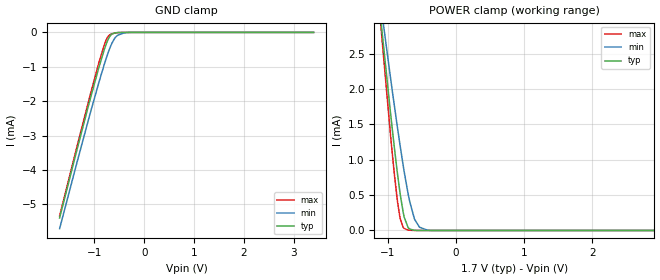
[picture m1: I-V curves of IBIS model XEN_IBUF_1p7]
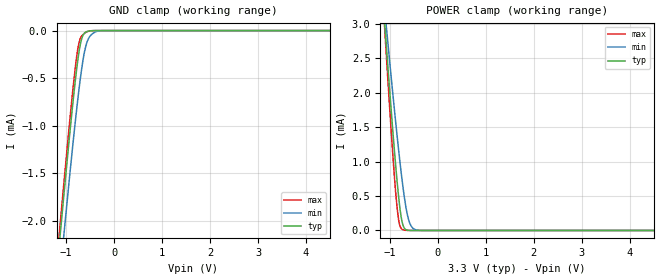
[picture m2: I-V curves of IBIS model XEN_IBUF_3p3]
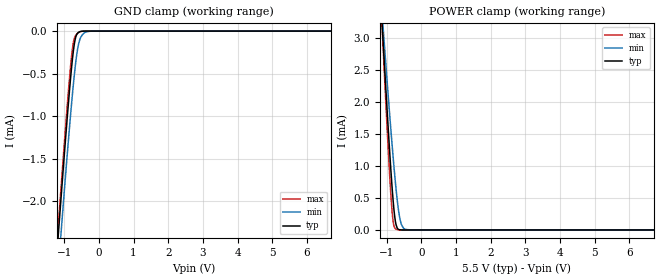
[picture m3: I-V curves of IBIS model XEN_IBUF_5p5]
|Texas Instruments Incorporated
| DAC874xH, HART & FOUNDATION Fieldbus / PROFIBUS PA Modems
| Device NAme#   Digital Voltage Range   Package-type   #pins
| DAC8740H   1.71V-5.5V   VQFN   24
| DAC8741H   1.71V-5.5V   VQFN   24
| DAC8742H   1.71V-5.5V   VQFP   32
[IBIS Ver]   4.1
[File name]   dac874xh.ibs
[Date]   02/17/2017
[File Rev]   1.0
[Source]
| Texas Instruments Incorporated.
| Analog-eLab Design Center, HPA
| 12500 TI Blvd
| Dallas, TX -75243
[Notes]   Revision History:
| Rev 1.0: 02/17/2017
| - Initial version of the model
| - Model generated from simulations in SPECTRE
| - Model matched to SPICE simulation
| - C_comp although listed in numerical order of value are
|   obtained from varying PVT conditions. For PVT conditions for
|   each specific value refer the buffer description under
|   respective [Model]. IBIS model user is responsible for using
|   appropriate C_comp to simulate for Signal Integrity.
[Disclaimer]
| This model is designed as an aid for customers of Texas Instruments.
| TI and its licensors and suppliers make no warranties, either expressed
| or implied, with respect to this  model, including the warranties of
| merchantability or fitness for a particular purpose. The model is
| provided solely on an "as is" basis. The entire risk as to its quality
| and performance is with the customer.
[Copyright]
(C) Copyright 2017 Texas Instruments Incorporated.All rights reserved.
|   DAC8740H
[Component]   DAC8740H
[Manufacturer]  TI
[Package]   |24 VQFN
|   typ   min   max
R_pkg   0.1   0.08   0.12
L_pkg   1.0nH   0.8nH   1.2nH
C_pkg   0.2pF   0.16pF   0.24pF
[Pin]  signal_name   model_name   R_pin   L_pin   C_pin
1   XEN   XEN_IBUF   NA   NA   NA
2   CLKO   CLKO_OBUF   NA   NA   NA
3   CLK_CFG0   CLK_CFG0_IBUF   NA   NA   NA
4   CLK_CFG1   XEN_IBUF   NA   NA   NA
5   RST   XEN_IBUF   NA   NA   NA
6   CD   CLKO_OBUF   NA   NA   NA
7   UART_IN   XEN_IBUF   NA   NA   NA
8   UART_RTS   SCLK_IBUF   NA   NA   NA
9   DUPLEX   XEN_IBUF   NA   NA   NA
10   UART_OUT   CLKO_OBUF   NA   NA   NA
11   IOVDD   power   NA   NA   NA
12   DGND   gnd   NA   NA   NA
13   REG_CAP   nc   NA   NA   NA
14   MOD_OUT   nc   NA   NA   NA
15   REF   nc   NA   NA   NA
16   MOD_IN   nc   NA   NA   NA
17   MOD_INF   nc   NA   NA   NA
18   AVDD   power   NA   NA   NA
19   AGND   gnd   NA   NA   NA
20   X2   nc   NA   NA   NA
21   X1   X1_IBUF   NA   NA   NA
22   DGND   gnd   NA   NA   NA
23   REF_EN   XEN_IBUF   NA   NA   NA
24   BPF_EN   XEN_IBUF   NA   NA   NA
|   DAC8741H
[Component]   DAC8741H
[Manufacturer]   TI
[Package]   |24 VQFN
|   typ   min   max
R_pkg   0.1   0.08   0.12
L_pkg   1.0nH   0.8nH   1.2nH
C_pkg   0.2pF   0.16pF   0.24pF
[Pin]  signal_name   model_name   R_pin   L_pin   C_pin
1   XEN   XEN_IBUF   NA   NA   NA
2   CLKO   CLKO_OBUF   NA   NA   NA
3   CLK_CFG0   CLK_CFG0_IBUF   NA   NA   NA
4   CLK_CFG1   XEN_IBUF   NA   NA   NA
5   RST   XEN_IBUF   NA   NA   NA
6   IRQ   CLKO_OBUF   NA   NA   NA
7   CS   XEN_IBUF   NA   NA   NA
8   SCLK   SCLK_IBUF   NA   NA   NA
9   SDI   XEN_IBUF   NA   NA   NA
10   SDO   CLKO_OBUF   NA   NA   NA
11   IOVDD   power   NA   NA   NA
12   DGND   gnd   NA   NA   NA
13   REG_CAP   nc   NA   NA   NA
14   MOD_OUT   nc   NA   NA   NA
15   REF   nc   NA   NA   NA
16   MOD_IN   nc   NA   NA   NA
17   MOD_INF   nc   NA   NA   NA
18   AVDD   power   NA   NA   NA
19   AGND   gnd   NA   NA   NA
20   X2   nc   NA   NA   NA
21   X1   X1_IBUF   NA   NA   NA
22   DGND   gnd   NA   NA   NA
23   REF_EN   XEN_IBUF   NA   NA   NA
24   BPF_EN   XEN_IBUF   NA   NA   NA
|   DAC8742H
[Component]   DAC8742H
[Manufacturer]   TI
[Package]   |32 VQFP
|   typ   min   max
R_pkg   0.1   0.08   0.12
L_pkg   1.0nH   0.8nH   1.2nH
C_pkg   0.2pF   0.16pF   0.24pF
[Pin]  signal_name   model_name   R_pin   L_pin   C_pin
1   NC   nc   NA   NA   NA
2   XEN   XEN_IBUF   NA   NA   NA
3   CLKO   CLKO_OBUF   NA   NA   NA
4   CLK_CFG0   CLK_CFG0_IBUF   NA   NA   NA
5   CLK_CFG1   XEN_IBUF   NA   NA   NA
6   RST   XEN_IBUF   NA   NA   NA
7   CD/IRQ   CLKO_OBUF   NA   NA   NA
8   NC   nc   NA   NA   NA
9   IF_SEL   IFSEL_IBUF   NA   NA   NA
10   UART_IN/CS   XEN_IBUF   NA   NA   NA
11   UART_RTS/SCLK   SCLK_IBUF   NA   NA   NA
12   DUPLEX/SDI   XEN_IBUF   NA   NA   NA
13   UART_OUT/SDO   CLKO_OBUF   NA   NA   NA
14   IOVDD   power   NA   NA   NA
15   DGND   gnd   NA   NA   NA
16   NC   nc   NA   NA   NA
17   NC   nc   NA   NA   NA
18   REG_CAP   nc   NA   NA   NA
19   MOD_OUT   nc   NA   NA   NA
20   REF   nc   NA   NA   NA
21   MOD_IN   nc   NA   NA   NA
22   MOD_INF   nc   NA   NA   NA
23   AVDD   power   NA   NA   NA
24   NC   nc   NA   NA   NA
25   NC   nc   NA   NA   NA
26   AGND   gnd   NA   NA   NA
27   X2   nc   NA   NA   NA
28   X1   X1_IBUF   NA   NA   NA
29   DGND   gnd   NA   NA   NA
30   REF_EN   XEN_IBUF   NA   NA   NA
31   BPF_EN   XEN_IBUF   NA   NA   NA
32   NC   nc   NA   NA   NA
|   Model Selectors
[Model Selector] XEN_IBUF
XEN_IBUF_1p7   1.7V  digital Input
XEN_IBUF_3p3   3.3V  digital Input
XEN_IBUF_5p5   5.5V  digital Input
[Model Selector] CLKO_OBUF
CLKO_OBUF_1p7   1.7V  digital Output
CLKO_OBUF_3p3   3.3V  digital Output
CLKO_OBUF_5p5   5.5V  digital Output
[Model Selector] CLK_CFG0_IBUF
CLK_CFG0_IBUF_1p7   1.7V  digital Input
CLK_CFG0_IBUF_3p3   3.3V  digital Input
CLK_CFG0_IBUF_5p5   5.5V  digital Input
[Model Selector] IFSEL_IBUF
IFSEL_IBUF_1p7   1.8V  digital Input
IFSEL_IBUF_3p3   3.3V  digital Input
IFSEL_IBUF_5p5   5.5V  digital Input
[Model Selector] SCLK_IBUF
SCLK_IBUF_1p7   1.7V  digital Input
SCLK_IBUF_3p3   3.3V  digital Input
SCLK_IBUF_5p5   5.5V  digital Input
[Model Selector] X1_IBUF
X1_IBUF_1p7   1.7V  analog Input
X1_IBUF_3p3   3.3V  analog Input
X1_IBUF_5p5   5.5V  analog Input
| Models and submodels in the file (18): XEN_IBUF_1p7 (Input), XEN_IBUF_3p3 (Input), XEN_IBUF_5p5 (Input), CLKO_OBUF_1p7 (3-state), CLKO_OBUF_3p3 (3-state), CLKO_OBUF_5p5 (3-state), CLK_CFG0_IBUF_1p7 (Input), CLK_CFG0_IBUF_3p3 (Input), CLK_CFG0_IBUF_5p5 (Input), IFSEL_IBUF_1p7 (Input), IFSEL_IBUF_3p3 (Input), IFSEL_IBUF_5p5 (Input), SCLK_IBUF_1p7 (Input), SCLK_IBUF_3p3 (Input), SCLK_IBUF_5p5 (Input), X1_IBUF_1p7 (Input), X1_IBUF_3p3 (Input), X1_IBUF_5p5 (Input)
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|   XEN_IBUF_1p7 Model
[Model]   XEN_IBUF_1p7
Model_type   Input
Vinl = 0.51
Vinh = 1.19
|   typ   min   max
C_comp   1.23E-13   1.77948E-14  2.05096E-13
| Where nom  PVT is Nominal Process, 1.7V, 27C
|   Fast PVT is Strong Process,  1.701V, -40C
|   Slow PVT is Weak Process,   1.699V, 150C
[Model spec]
|subparameter
Vinl   0.51   0.5097   0.5103
Vinh   1.19   1.1893   1.1907
[Voltage Range]   1.7   1.699   1.701
[Temperature Range]   27   150   -40
[Power Clamp Reference]   1.7   1.699   1.701
[GND Clamp Reference]   0   0   0
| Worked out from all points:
|   GND clamp passes 1 mA (typ) near -0.91 V on its own axis
|   POWER clamp passes 1 mA (typ) near -0.89 V on its own axis
[GND Clamp]
|   Voltage   I(typ)   I(min)   I(max)
-1.7V     -5.395mA   -5.705mA   -5.337mA
-1.348V   -3.396mA   -3.765mA   -3.303mA
-1.088V   -1.954mA   -2.366mA   -1.834mA
-914.6mV  -1.037mA   -1.472mA   -898.7uA
-802.4mV  -500.1uA   -929.6uA   -361.7uA
-741.2mV  -257.3uA   -658.1uA   -150.9uA
-685.1mV  -103.7uA   -436.3uA   -64.18uA
-603.5mV  -20.82uA   -192.8uA   -23.73uA
-532.1mV  -4.942uA   -82.74uA   -6.847uA
-419.9mV  -262.1nA   -22.06uA   -297.3nA
-261.8mV  0A         -823.5nA   0A
3.4V      0A         0A         0A
[POWER Clamp]
|   Voltage   I(typ)   I(min)   I(max)
-1.7V     8.86mA     7.737mA    9.912mA
-1.098V   2.909mA    3.136mA    2.814mA
-965.6mV  1.682mA    2.174mA    1.371mA
-909.5mV  1.194mA    1.781mA    819.5uA
-868.7mV  860.8uA    1.503mA    469.3uA
-817.7mV  489.8uA    1.168mA    154.7uA
-761.6mV  185.6uA    823.9uA    27.95uA
-705.5mV  41.46uA    519.2uA    6.332uA
-608.6mV  1.632uA    154.1uA    500.9nA
-537.2mV  145.1nA    45.24uA    47.67nA
-419.9mV  0A         3.894uA    0A
3.4V      0A         0A         0A
|   XEN_IBUF_3p3 Model
[Model]   XEN_IBUF_3p3
Model_type   Input
Vinl = 0.99
Vinh = 2.31
|   typ   min   max
C_comp   1.45175E-13  3.60452E-14   2.15954E-13
| Where nom  PVT is Nominal Process, 3.3V, 27C
|   Fast PVT is Strong Process,  3.6V, -40C
|   Slow PVT is Weak Process,   3.0V, 150C
[Model spec]
|subparameter
Vinl   0.99   0.9   1.08
Vinh   2.31   2.1   2.52
[Voltage Range]   3.3   3   3.6
[Temperature Range]   27   150   -40
[Power Clamp Reference]   3.3   3   3.6
[GND Clamp Reference]   0   0   0
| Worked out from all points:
|   GND clamp passes 1 mA (typ) near -0.91 V on its own axis
|   POWER clamp passes 1 mA (typ) near -0.89 V on its own axis
[GND Clamp]
|   Voltage   I(typ)   I(min)   I(max)
-3.3V     -14.66mA   -14.73mA   -14.82mA
-1.251V   -2.851mA   -3.236mA   -2.747mA
-1.102V   -2.031mA   -2.441mA   -1.912mA
-1.053V   -1.763mA   -2.181mA   -1.639mA
-904.2mV  -984.9uA   -1.42mA    -845.2uA
-775.5mV  -386.5uA   -807.4uA   -256.6uA
-726mV    -207.6uA   -594.9uA   -117.3uA
-676.5mV  -87.92uA   -405.4uA   -57.67uA
-567.6mV  -10.36uA   -126uA     -13.56uA
-458.7mV  -1.404uA   -35.96uA   -1.048uA
-260.7mV  0A         -793.1nA   0A
6.6V      0A         0A         0A
[POWER Clamp]
|   Voltage   I(typ)   I(min)   I(max)
-3.3V     25.21mA    20.41mA    29.38mA
-1.112V   3.041mA    3.239mA    2.971mA
-1.092V   2.853mA    3.092mA    2.748mA
-1.023V   2.204mA    2.586mA    1.98mA
-933.9mV  1.402mA    1.95mA     1.052mA
-874.5mV  906.6uA    1.542mA    515.1uA
-805.2mV  410.3uA    1.089mA    107.9uA
-726mV    76.03uA    624.7uA    10.54uA
-656.7mV  8.383uA    304uA      1.865uA
-587.4mV  789.7nA    109.2uA    259.8nA
-399.3mV  0A         2.321uA    0A
6.6V      0A         0A         0A
|   XEN_IBUF_5p5 Model
[Model]   XEN_IBUF_5p5
Model_type   Input
Vinl = 1.65
Vinh = 3.85
|   typ   min   max
C_comp   1.62855E-13   6.2518E-14   2.17E-13
| Where nom  PVT is Nominal Process, 5.5V, 27C
|   Fast PVT is Strong Process,  5.501V, -40C
|   Slow PVT is Weak Process,   5.499V, 150C
[Model spec]
|subparameter
Vinl   1.65   1.6497   1.6503
Vinh   3.85   3.8493   3.8507
[Voltage Range]   5.5   5.499   5.501
[Temperature Range]   27   150   -40
[Power Clamp Reference]   5.5   5.499   5.501
[GND Clamp Reference]   0   0   0
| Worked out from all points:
|   GND clamp passes 1 mA (typ) near -0.91 V on its own axis
|   POWER clamp passes 1 mA (typ) near -0.89 V on its own axis
[GND Clamp]
|   Voltage   I(typ)   I(min)   I(max)
-5.5V     -27.53mA   -27.33mA   -27.99mA
-1.359V   -3.455mA   -3.822mA   -3.362mA
-1.177V   -2.442mA   -2.84mA    -2.331mA
-1.161V   -2.351mA   -2.751mA   -2.238mA
-1.127V   -2.17mA    -2.576mA   -2.053mA
-1.028V   -1.633mA   -2.054mA   -1.506mA
-880mV    -864.2uA   -1.3mA     -722.9uA
-781mV    -409uA     -832uA     -276.7uA
-682mV    -97.74uA   -425uA     -61.7uA
-550mV    -7.231uA   -102.1uA   -9.823uA
-203.5mV  0A         -151.1nA   0A
11V       0A         0A         0A
[POWER Clamp]
|   Voltage   I(typ)   I(min)   I(max)
-5.5V     48.9mA     43.04mA    56.37mA
-1.127V   3.188mA    3.353mA    3.146mA
-1.095V   2.874mA    3.109mA    2.773mA
-929.5mV  1.364mA    1.92mA     1.009mA
-847mV    695.3uA    1.358mA    313.7uA
-814mV    465.7uA    1.144mA    139.5uA
-764.5mV  197.6uA    840.9uA    30.47uA
-698.5mV  33.3uA     485uA      5.32uA
-632.5mV  3.669uA    220.1uA    970.2nA
-566.5mV  379nA      76.34uA    123.2nA
-302.5mV  0A         158.9nA    0A
11V       0A         0A         0A
